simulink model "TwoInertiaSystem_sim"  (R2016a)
settings: Solver=FixedStepAuto  StartTime=0.0  StopTime=Endtime  FixedStep=1e-3  RelTol=1e-3
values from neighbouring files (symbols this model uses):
  D_1 = 1e-2    (= 0.01)    [TwoInertiaSystem.m]
  D_2 = 2e-2    (= 0.02)    [TwoInertiaSystem.m]
  J_1 = 1e-2    (= 0.01)    [TwoInertiaSystem.m]
  J_2 = 2e-2    (= 0.02)    [TwoInertiaSystem.m]
  K = 0.1    [TwoInertiaSystem.m]    (also in Test2_1.m = 2)
  tau_1 = 1    [TwoInertiaSystem.m]
  tau_2 = -1    [TwoInertiaSystem.m]

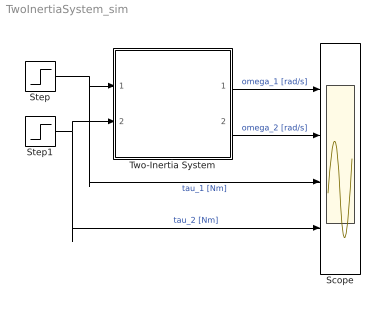
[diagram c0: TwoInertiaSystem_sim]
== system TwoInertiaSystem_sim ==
  Scope : Scope  NumInputPorts=4
  Step : Step  After=tau_1  SampleTime=0
  Step1 : Step  Time=10  After=tau_2  SampleTime=0
  Two-Inertia System : Subsystem
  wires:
  Step1/1 -> Scope/4, Two-Inertia System/2(tau_2 [Nm])  "tau_2 [Nm]"
  Two-Inertia System/1(omega_1 [rad/s]) -> Scope/1  "omega_1 [rad/s]"
  Two-Inertia System/2(omega_2 [rad/s]) -> Scope/2  "omega_2 [rad/s]"
  Step/1 -> Scope/3, Two-Inertia System/1(tau_1 [Nm])  "tau_1 [Nm]"

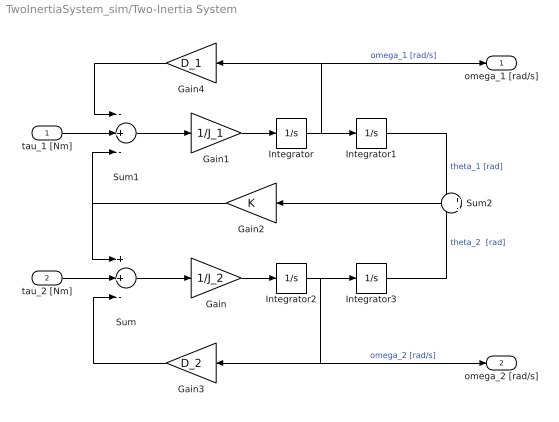
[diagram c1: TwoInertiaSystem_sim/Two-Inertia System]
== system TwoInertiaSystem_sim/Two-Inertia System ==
  tau_1 [Nm] : Inport
  tau_2 [Nm] : Inport  Port=2
  Gain : Gain  Gain=1/J_2
  Gain1 : Gain  Gain=1/J_1
  Gain2 : Gain  Gain=K
  Gain3 : Gain  Gain=D_2
  Gain4 : Gain  Gain=D_1
  Integrator{,1..3} (4 alike) : Integrator
  Sum : Sum  Inputs=++-
  Sum1 : Sum  Inputs=-+-
  Sum2 : Sum  Inputs=+|-
  omega_1 [rad/s] : Outport
  omega_2 [rad/s] : Outport  Port=2
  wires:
  tau_1 [Nm]/1 -> Sum1/2
  tau_2 [Nm]/1 -> Sum/2
  Integrator/1 -> Integrator1/1, omega_1 [rad/s]/1, Gain4/1  "omega_1 [rad/s]"
  Gain1/1 -> Integrator/1
  Sum1/1 -> Gain1/1
  Gain2/1 -> Sum1/3, Sum/1
  Integrator3/1 -> Sum2/2  "theta_2  [rad]"
  Integrator2/1 -> Integrator3/1, omega_2 [rad/s]/1, Gain3/1  "omega_2 [rad/s]"
  Gain/1 -> Integrator2/1
  Gain3/1 -> Sum/3
  Gain4/1 -> Sum1/1
  Sum/1 -> Gain/1
  Sum2/1 -> Gain2/1
  Integrator1/1 -> Sum2/1  "theta_1 [rad]"
